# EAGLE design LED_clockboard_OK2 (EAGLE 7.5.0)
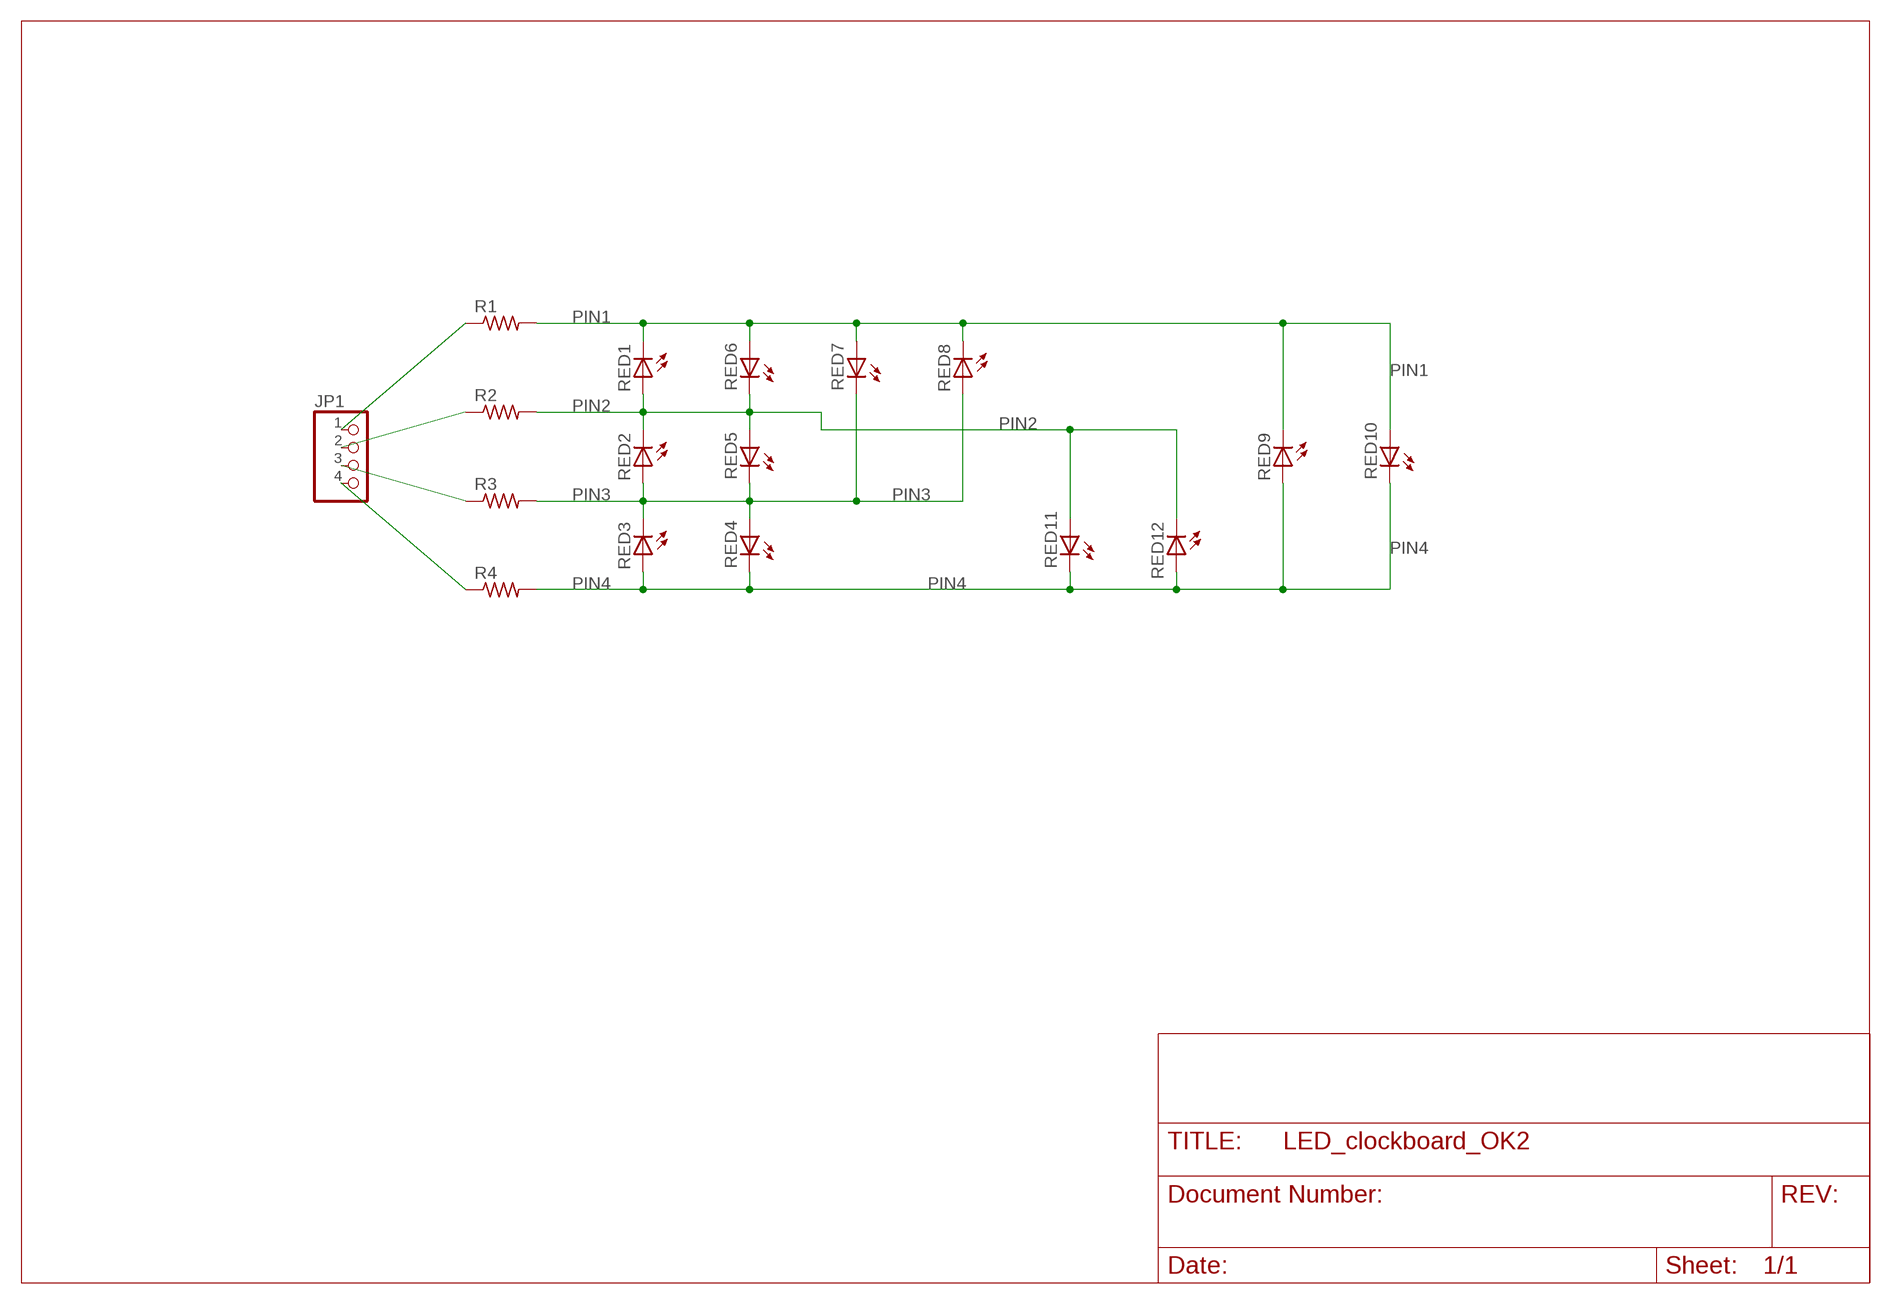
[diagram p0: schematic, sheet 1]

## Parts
JP1  PINHD-1X4  [1X04]
R1  RES-US1206FAB  [R1206FAB]
R2  RES-US1206FAB  [R1206FAB]
R3  RES-US1206FAB  [R1206FAB]
R4  RES-US1206FAB  [R1206FAB]
RED1  LEDFAB1206  [LED1206FAB]
RED2  LEDFAB1206  [LED1206FAB]
RED3  LEDFAB1206  [LED1206FAB]
RED4  LEDFAB1206  [LED1206FAB]
RED5  LEDFAB1206  [LED1206FAB]
RED6  LEDFAB1206  [LED1206FAB]
RED7  LEDFAB1206  [LED1206FAB]
RED8  LEDFAB1206  [LED1206FAB]
RED9  LEDFAB1206  [LED1206FAB]
RED10  LEDFAB1206  [LED1206FAB]
RED11  LEDFAB1206  [LED1206FAB]
RED12  LEDFAB1206  [LED1206FAB]

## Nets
N$2: JP1.1 R1.1
N$3: JP1.2 R2.1
N$4: JP1.3 R3.1
N$5: JP1.4 R4.1
PIN1: R1.2 RED1.2(C) RED6.1(A) RED7.1(A) RED8.2(C) RED9.2(C) RED10.1(A)
PIN2: R2.2 RED1.1(A) RED2.2(C) RED5.1(A) RED6.2(C) RED11.1(A) RED12.2(C)
PIN3: R3.2 RED2.1(A) RED3.2(C) RED4.1(A) RED5.2(C) RED7.2(C) RED8.1(A)
PIN4: R4.2 RED3.1(A) RED4.2(C) RED9.1(A) RED10.2(C) RED11.2(C) RED12.1(A)

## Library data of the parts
JP1 = pinhead:PINHD-1X4: PIN HEADER
R1-R4 = fab:RES-US: Resistor (US Symbol)
RED1-RED12 = fab:LED: LED

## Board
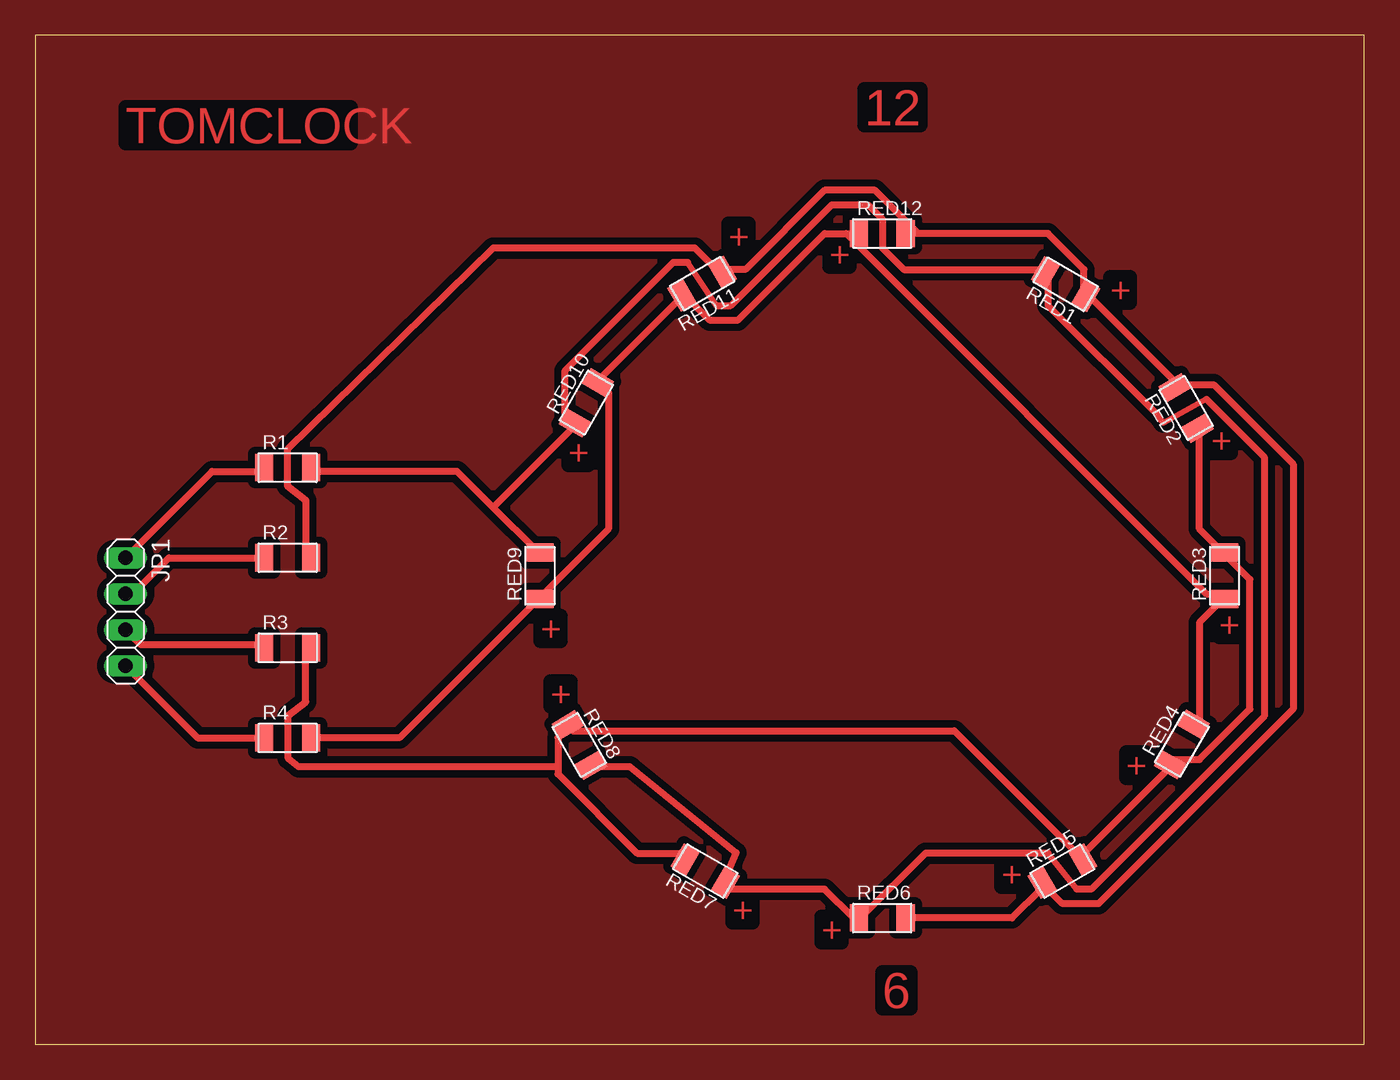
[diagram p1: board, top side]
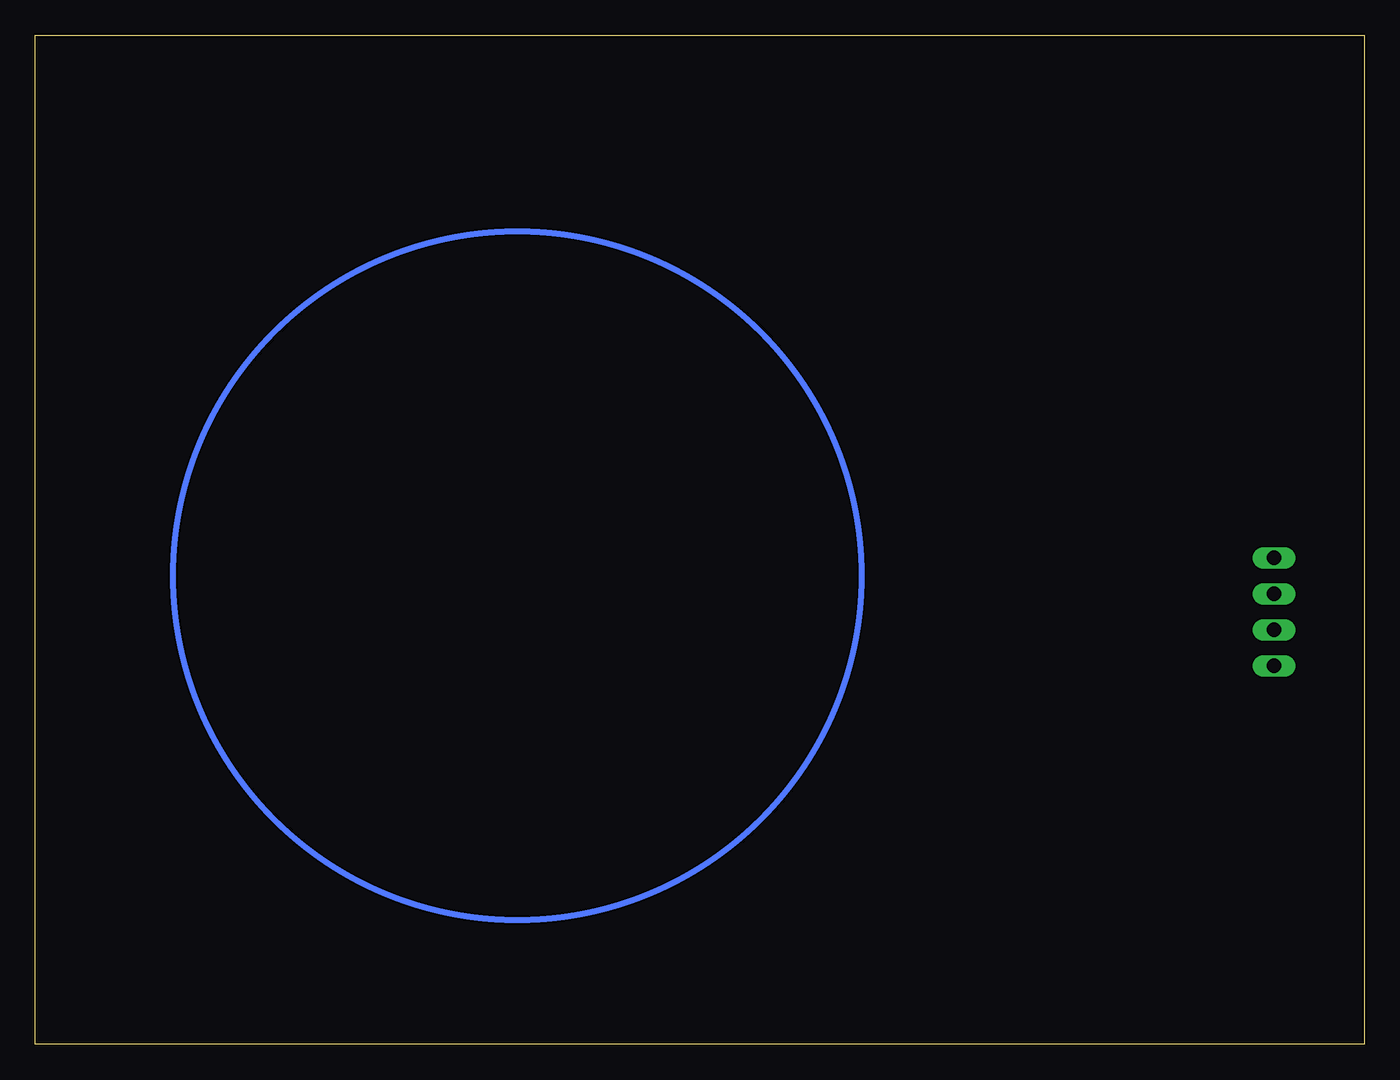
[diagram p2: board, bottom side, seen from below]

Size 93.65 x 71.11 mm. Coordinates in mm from the lower left corner, seen from the top.
Outline: 0,0 93.65,0 93.65,71.11 0,71.11 0,0
Copper layers (1*16): Top 0.035mm / dielectric 1.5mm / Bottom 0.035mm
Design rules "default *": minimum track width 20mil, minimum drill 24mil, track to track 20mil, track to pad 20mil, pad to pad 8mil, via to via 8mil, smd to smd 8mil, copper to edge 0mil, drill to drill 8mil, minimum pad ring 10mil, minimum via ring 8mil, stop-mask expansion 4mil, vias tented up to drill 0mil, thermal gap 10mil

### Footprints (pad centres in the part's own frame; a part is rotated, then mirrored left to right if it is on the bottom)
1X04 = drill 1.016 long: 1 -3.81,0; 2 -1.27,0; 3 1.27,0; 4 3.81,0
R1206FAB = smd 1.27 x 1.905: 1 -1.651,0; 2 1.651,0
LED1206FAB = smd 1.27 x 1.905: 1 -1.651,0; 2 1.651,0

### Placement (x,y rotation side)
JP1  6.35,30.48 270 top
R1  17.78,40.64 0 top
R2  17.78,34.29 0 top
R3  17.78,27.94 0 top
R4  17.78,21.59 0 top
RED1  72.62,53.57 150 top
RED2  81.11,44.85 120 top
RED3  83.82,33.02 90 top
RED4  80.82,21.13 60 top
RED5  72.39,12.2 30 top
RED6  59.69,8.89 0 top
RED7  47.22,12.2 150 top
RED8  38.33,21.09 300 top
RED9  35.56,33.02 90 top
RED10  38.83,45.22 60 top
RED11  46.99,53.61 210 top
RED12  59.69,57.15 0 top

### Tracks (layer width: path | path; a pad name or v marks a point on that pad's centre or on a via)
N$1
  pour Top: -3.81,74.93 97.79,74.93 97.79,-5.08 -3.81,-5.08
N$2
  Top 0.508: JP1.1 12.45,40.39 16,40.39 R1.1
N$3
  Top 0.508: R2.1 9.4,34.29 6.86,31.75 JP1.2
N$4
  Top 0.508: JP1.3 7.37,28.19 16,28.19 R3.1
N$5
  Top 0.508: R4.1 11.43,21.59 JP1.4
PIN1
  Top 0.406: 73.41,10.92 71.37,13.46 | 82.55,45.47 79.49,43.8 78.99,44.45 | 48.01,52.07 45.97,55.12
  Top 0.508: RED8.2 39.37,19.56 41.91,19.56 49.39,13.5 48.51,11.43 RED7.1 49.02,10.92 55.63,10.92 57.66,8.89 RED6.1 58.17,8.89 62.74,13.46 71.37,13.46 | 32.26,37.85 35.31,34.8 RED9.2 | 32.26,37.85 29.72,40.39 19.56,40.39 R1.2 | 32.26,37.85 37.85,43.43 RED10.1 37.85,43.94 37.34,44.45 37.34,47.5 44.96,55.12 45.97,55.12 | 48.01,52.07 49.02,52.07 56.13,59.18 58.67,59.18 59.69,58.17 59.69,56.13 61.21,54.61 70.87,54.61 RED1.2 71.37,54.1 71.37,52.07 78.99,44.45 | 73.41,10.92 74.42,10.92 86.61,23.11 86.61,41.4 82.55,45.47
PIN2
  Top 0.508: R2.2 19.05,34.29 19.05,38.35 17.74,39.37 17.74,41.91 32.26,56.13 46.48,56.13 48.01,54.61 RED11.1 48.51,54.61 50.04,54.61 55.63,60.2 59.18,60.2 62.23,57.15 | RED6.2 68.83,8.89 70.87,10.92 RED5.1 71.37,10.92 72.39,9.91 74.93,9.91 88.65,23.62 88.65,40.89 83.06,46.48 80.52,46.48 | 80.52,46.48 74.42,52.58 RED1.1 73.91,53.09 73.91,54.61 71.37,57.15 62.23,57.15 | 62.23,57.15 RED12.2 | 80.52,46.48 RED2.2
PIN3
  Top 0.508: RED2.1 82.04,42.93 82.04,36.32 83.57,34.8 RED3.2 84.07,34.29 85.6,32.77 85.6,23.62 82.04,20.07 80.01,20.07 RED4.1 80.01,19.56 73.91,13.46 RED5.2 73.41,13.46 64.77,22.1 37.85,22.1 RED8.1 37.34,22.1 36.83,21.59 36.83,19.56 | 36.83,19.56 36.83,19.05 42.42,13.46 45.47,13.46 RED7.2 | 36.83,19.56 18.54,19.56 17.82,20.14 17.82,23.19 19.05,24.13 19.05,27.69 R3.2
PIN4
  Top 0.508: R4.2 25.65,21.59 35.31,31.24 RED9.1 35.81,31.75 40.39,36.32 40.39,45.97 39.88,46.48 RED10.2 39.88,46.99 45.47,52.58 RED11.2 45.97,52.58 47.5,51.05 49.53,51.05 55.63,57.15 57.15,57.15 | RED4.2 82.04,22.61 82.04,29.72 83.57,31.24 RED3.1 83.57,31.75 82.55,31.75 57.15,57.15 | 57.15,57.15 RED12.1
(copper drawn outside any net)
  shapes: Bottom circle x1

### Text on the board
Top: 12 | TOMCLOCK | + | + | + | + | + | + | + | + | + | + | + | + | 6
